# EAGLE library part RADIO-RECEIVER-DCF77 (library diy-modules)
DCF-77 Longwave Radio Time Signal Receiver based on MAS6180B1 chip
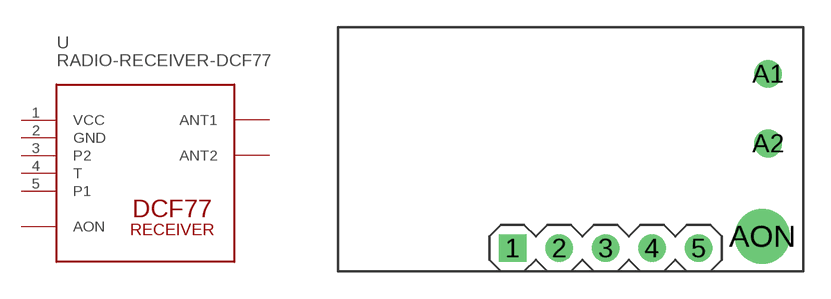
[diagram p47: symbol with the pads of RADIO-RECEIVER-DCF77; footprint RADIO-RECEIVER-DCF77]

Designator prefix -

## RADIO-RECEIVER-DCF77  [RADIO-RECEIVER-DCF77]
1  VCC  pwr
2  GND  pwr
3  P2
4  T  out
5  P1
A1  ANT1  pas
A2  ANT2  pas
AON  AON

## Footprint RADIO-RECEIVER-DCF77 (pad centres in mm)
DCF-77 Longwave Radio Time Signal Receiver based on MAS6180B1 chip
drill 1 square: 1 -3.175,-5.08
drill 1: 2 -0.635,-5.08; 3 1.905,-5.08; 4 4.445,-5.08; 5 6.985,-5.08; A1 10.795,4.445; A2 10.795,0.635
drill 2: AON 10.477,-4.445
